(* Logix 5000 Rung export; software revision 16.04; part 2 of 2 *)
(* AOI56EAFC, continued *)

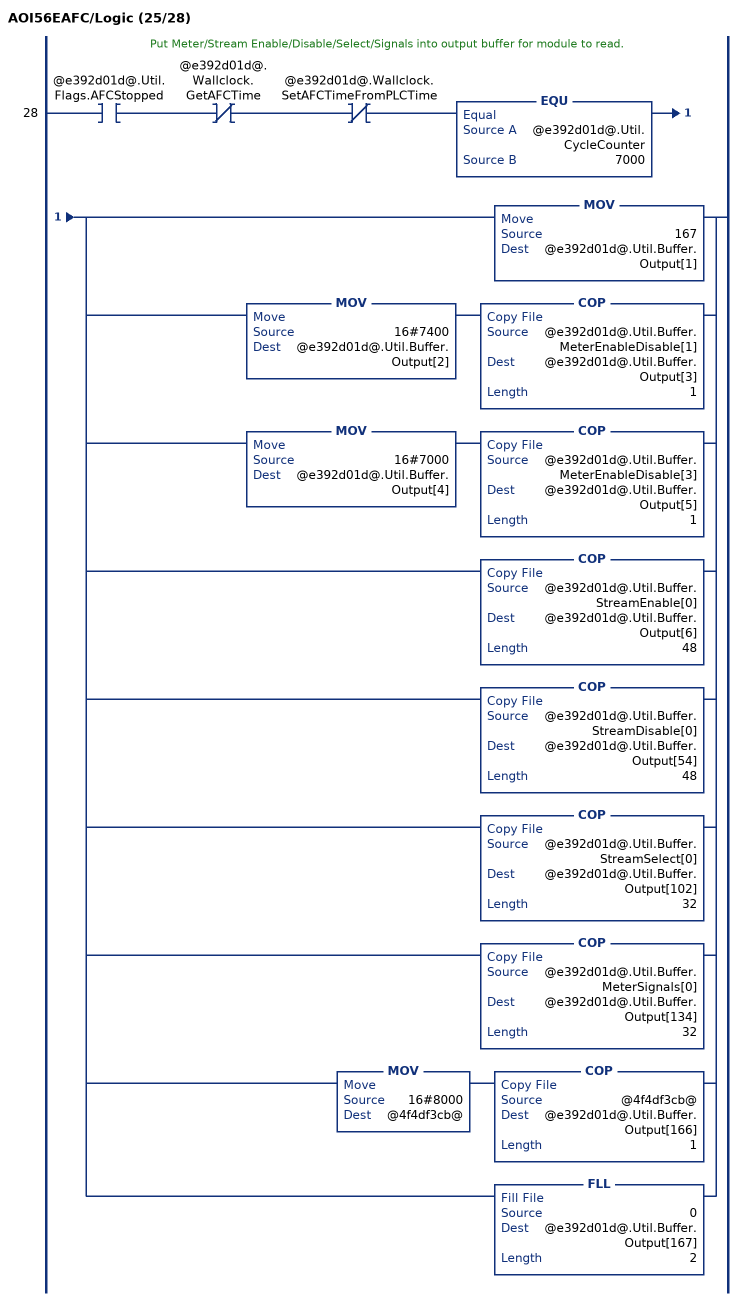
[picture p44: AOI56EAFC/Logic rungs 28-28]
   // Put Meter/Stream Enable/Disable/Select/Signals into output buffer for module to read.
   28: XIC(@e392d01d@.Util.Flags.AFCStopped)XIO(@e392d01d@.Wallclock.GetAFCTime)XIO(@e392d01d@.Wallclock.SetAFCTimeFromPLCTime)EQU(@e392d01d@.Util.CycleCounter,7000)[MOV(167,@e392d01d@.Util.Buffer.Output[1]) ,MOV(16#7400,@e392d01d@.Util.Buffer.Output[2]) COP(@e392d01d@.Util.Buffer.MeterEnableDisable[1],@e392d01d@.Util.Buffer.Output[3],1) ,MOV(16#7000,@e392d01d@.Util.Buffer.Output[4]) COP(@e392d01d@.Util.Buffer.MeterEnableDisable[3],@e392d01d@.Util.Buffer.Output[5],1) ,COP(@e392d01d@.Util.Buffer.StreamEnable[0],@e392d01d@.Util.Buffer.Output[6],48) ,COP(@e392d01d@.Util.Buffer.StreamDisable[0],@e392d01d@.Util.Buffer.Output[54],48) ,COP(@e392d01d@.Util.Buffer.StreamSelect[0],@e392d01d@.Util.Buffer.Output[102],32) ,COP(@e392d01d@.Util.Buffer.MeterSignals[0],@e392d01d@.Util.Buffer.Output[134],32) ,[MOV(16#8000,@4f4df3cb@) COP(@4f4df3cb@,@e392d01d@.Util.Buffer.Output[166],1) ,FLL(0,@e392d01d@.Util.Buffer.Output[167],2) ] ];
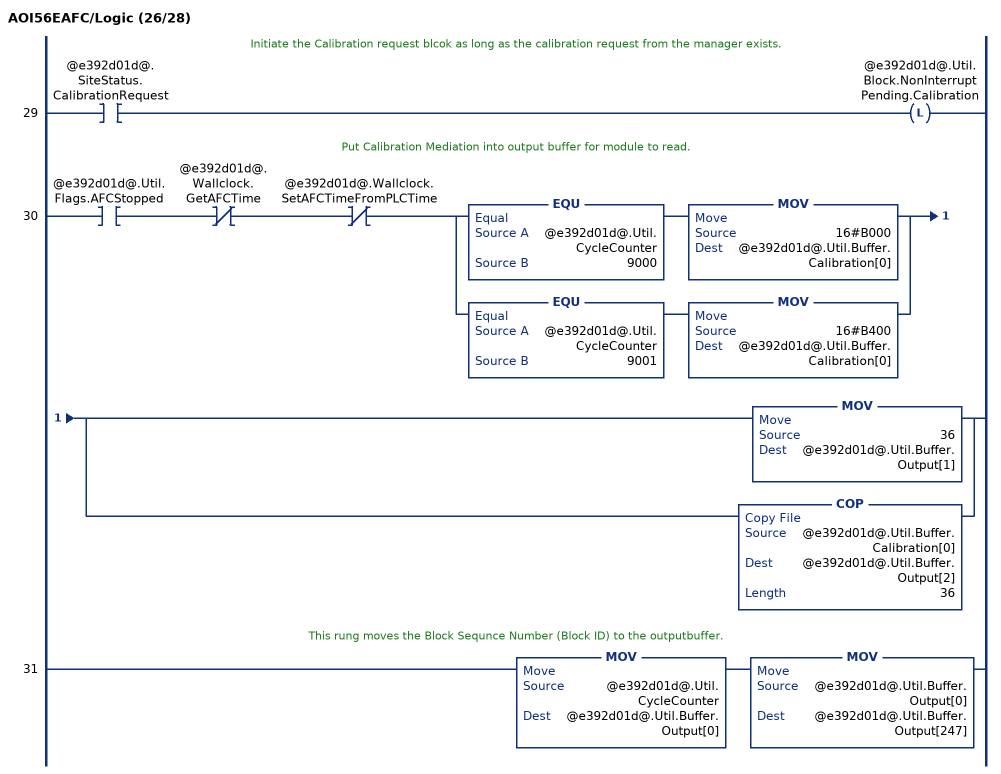
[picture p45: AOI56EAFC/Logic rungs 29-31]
   // Initiate the Calibration request blcok as long as the calibration request from the manager exists.
   29: XIC(@e392d01d@.SiteStatus.CalibrationRequest)OTL(@e392d01d@.Util.Block.NonInterruptPending.Calibration);
   // Put Calibration Mediation into output buffer for module to read.
   30: XIC(@e392d01d@.Util.Flags.AFCStopped)XIO(@e392d01d@.Wallclock.GetAFCTime)XIO(@e392d01d@.Wallclock.SetAFCTimeFromPLCTime)[EQU(@e392d01d@.Util.CycleCounter,9000) MOV(16#B000,@e392d01d@.Util.Buffer.Calibration[0]) ,EQU(@e392d01d@.Util.CycleCounter,9001) MOV(16#B400,@e392d01d@.Util.Buffer.Calibration[0]) ][MOV(36,@e392d01d@.Util.Buffer.Output[1]) ,COP(@e392d01d@.Util.Buffer.Calibration[0],@e392d01d@.Util.Buffer.Output[2],36) ];
   // This rung moves the Block Sequnce Number (Block ID) to the outputbuffer.
   31: MOV(@e392d01d@.Util.CycleCounter,@e392d01d@.Util.Buffer.Output[0])MOV(@e392d01d@.Util.Buffer.Output[0],@e392d01d@.Util.Buffer.Output[247]);
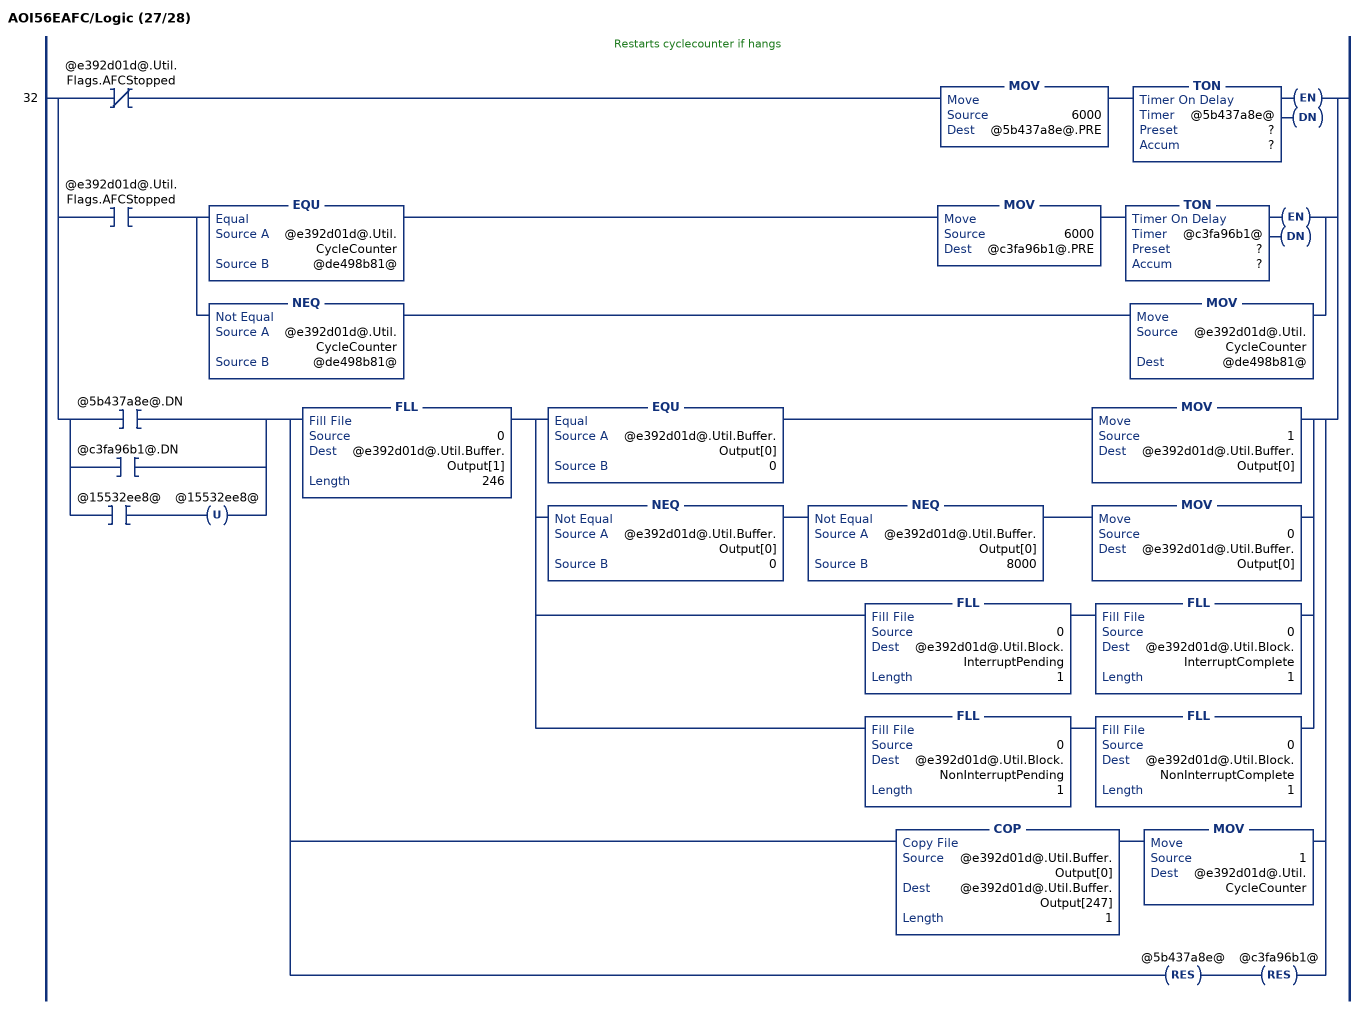
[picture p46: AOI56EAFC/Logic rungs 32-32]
   // Restarts cyclecounter if hangs
   32: [XIO(@e392d01d@.Util.Flags.AFCStopped) MOV(6000,@5b437a8e@.PRE) TON(@5b437a8e@,?,?) ,XIC(@e392d01d@.Util.Flags.AFCStopped) [EQU(@e392d01d@.Util.CycleCounter,@de498b81@) MOV(6000,@c3fa96b1@.PRE) TON(@c3fa96b1@,?,?) ,NEQ(@e392d01d@.Util.CycleCounter,@de498b81@) MOV(@e392d01d@.Util.CycleCounter,@de498b81@) ] ,[[XIC(@5b437a8e@.DN) ,XIC(@c3fa96b1@.DN) ] ,XIC(@15532ee8@) OTU(@15532ee8@) ] [FLL(0,@e392d01d@.Util.Buffer.Output[1],246) [EQU(@e392d01d@.Util.Buffer.Output[0],0) MOV(1,@e392d01d@.Util.Buffer.Output[0]) ,NEQ(@e392d01d@.Util.Buffer.Output[0],0) NEQ(@e392d01d@.Util.Buffer.Output[0],8000) MOV(0,@e392d01d@.Util.Buffer.Output[0]) ,FLL(0,@e392d01d@.Util.Block.InterruptPending,1) FLL(0,@e392d01d@.Util.Block.InterruptComplete,1) ,FLL(0,@e392d01d@.Util.Block.NonInterruptPending,1) FLL(0,@e392d01d@.Util.Block.NonInterruptComplete,1) ] ,COP(@e392d01d@.Util.Buffer.Output[0],@e392d01d@.Util.Buffer.Output[247],1) MOV(1,@e392d01d@.Util.CycleCounter) ,RES(@5b437a8e@) RES(@c3fa96b1@) ] ];
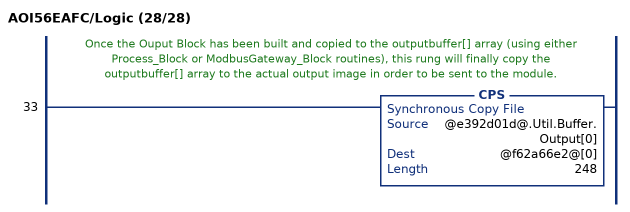
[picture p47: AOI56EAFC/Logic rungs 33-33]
   // Once the Ouput Block has been built and copied to the outputbuffer[] array (using either Process_Block or ModbusGateway_Block routines), this rung will finally copy the outputbuffer[] array to the actual output image in order to be sent to the module.
   33: CPS(@e392d01d@.Util.Buffer.Output[0],@f62a66e2@[0],248);
END_ROUTINE

ROUTINE Prescan   (* ladder *)
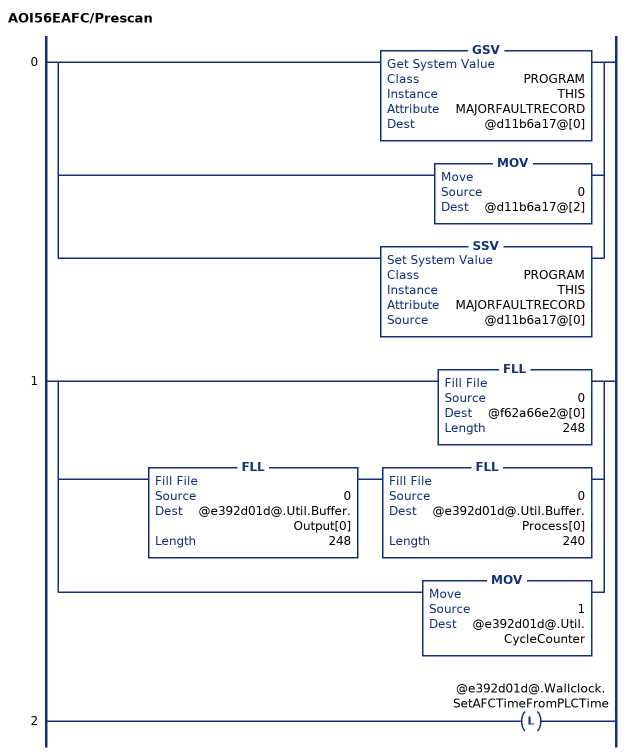
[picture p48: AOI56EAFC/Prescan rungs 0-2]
   0: [GSV(PROGRAM,THIS,MAJORFAULTRECORD,@d11b6a17@[0]) ,MOV(0,@d11b6a17@[2]) ,SSV(PROGRAM,THIS,MAJORFAULTRECORD,@d11b6a17@[0]) ];
   1: [FLL(0,@f62a66e2@[0],248) ,FLL(0,@e392d01d@.Util.Buffer.Output[0],248) FLL(0,@e392d01d@.Util.Buffer.Process[0],240) ,MOV(1,@e392d01d@.Util.CycleCounter) ];
   2: OTL(@e392d01d@.Wallclock.SetAFCTimeFromPLCTime);
END_ROUTINE
END_ADD_ON_INSTRUCTION

VAR_GLOBAL   (* controller tags *)
   AFC : AFCEModuleDef;
   Local:1:I : AB:1756_MODULE_INT_500Bytes:I:0;
   AOI56EAFC : AOI56EAFC;
   Local:1:O : AB:1756_MODULE_INT_496Bytes:O:0;
END_VAR

PROGRAM MainProgram

ROUTINE MainRoutine   (* ladder *)
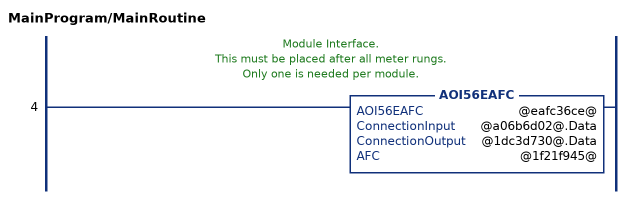
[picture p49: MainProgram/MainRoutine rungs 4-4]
   // Module Interface.
   // This must be placed after all meter rungs.
   // Only one is needed per module.
   4: AOI56EAFC(@eafc36ce@,@a06b6d02@.Data,@1dc3d730@.Data,@1f21f945@);
END_ROUTINE
END_PROGRAM
